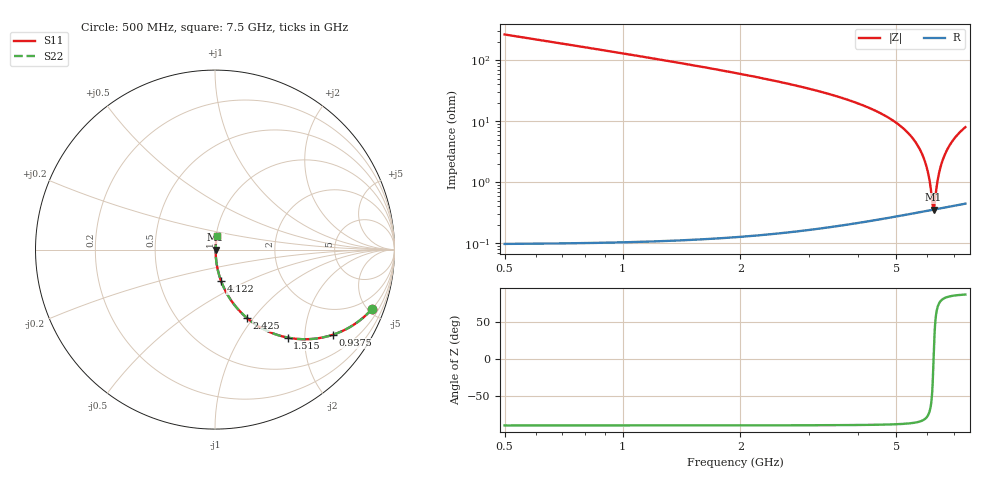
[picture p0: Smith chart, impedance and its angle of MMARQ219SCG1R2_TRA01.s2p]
! MMARQ219SCG1R2_TRA01  S-PARAMETER MODEL  ( General Type )
! Model Generated by TAIYO YUDEN Corporation (http://www.ty-top.com)
! Version 1.0
! TAIYO YUDEN Control No. 180601
! Copyright(c) 2018 TAIYO YUDEN CO.,LTD. All Rights Reserved.
! Product Description (link to TY-COMPAS)
! https://ds.yuden.co.jp/TYCOMPAS/or/detail?pn=MMARQ219SCG1R2BTRA01&u=M
! Products Name : Multilayer Ceramic Capacitors
! Characteristics :
!  Capacitance : 1.2 pF , Rated Voltage : 250V , TCC : CG / C0G
!  Case Size : 2.0 x 1.25 / 0.079 x 0.049 [mm/inch] , Thickness : 0.85 / 0.033 [mm/inch]
!  (Conditions: Temperature = 25 degC , DC Bias Current/Voltage = 0A / 0V)
! External Node Assignments :
!  1  o---| |---o  2
! GND o---------o GND
! Frequency Range : 500MHz  -  7500MHz  [ 401 STEP ]
# MHz S RI R 50
! Freq[MHz].  S11 Real  S11 Imag  S21 Real  S21 Imag  S12 Real  S12 Imag  S22 Real  S22 Imag
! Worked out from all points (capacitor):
!   401 points, 500 MHz to 7.5 GHz, reference 50 ohm
!   read as one part in series: C = 1.2 pF near 535 MHz
!   lowest |Z| = 354 mohm at 6.223 GHz (marker M1)
!   series resonance near 6.222 GHz, so ESL is about 550 pH
!   S11 on the Smith chart (normalised r, x): 500 MHz: 1.00, -5.27; 937.5 MHz: 1.00, -2.76; 1.515 GHz: 1.00, -1.65; 2.425 GHz: 1.00, -0.93; 4.122 GHz: 1.00, -0.36; 7.5 GHz: 1.01, +0.16
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500  0.874 -0.3316  0.126 0.3316  0.126 0.3316  0.874 -0.3316
937.5  0.6564 -0.4745  0.3436 0.4745  0.3436 0.4745  0.6564 -0.4745
1515  0.4041 -0.49  0.5959 0.49  0.5959 0.49  0.4041 -0.49
1672.5  0.3512 -0.4766  0.6488 0.4766  0.6488 0.4766  0.3512 -0.4766
2425  0.1776 -0.3806  0.8224 0.3806  0.8224 0.3806  0.1776 -0.3806
2845  0.1205 -0.3234  0.8795 0.3234  0.8795 0.3234  0.1205 -0.3234
4000  0.0382 -0.1863  0.9618 0.1863  0.9618 0.1863  0.0382 -0.1863
4122.5  0.0334 -0.1737  0.9666 0.1737  0.9666 0.1737  0.0334 -0.1737
5172.5  0.00897 -0.078  0.991 0.078  0.991 0.078  0.00897 -0.078
5592.5  0.00514 -0.045  0.9949 0.045  0.9949 0.045  0.00514 -0.045
5872.5  0.00389 -0.0243  0.9961 0.0243  0.9961 0.0243  0.00389 -0.0243
6047.5  0.00356 -0.012  0.9964 0.012  0.9964 0.012  0.00356 -0.012
6100  0.00352 -0.00831  0.9965 0.00831  0.9965 0.00831  0.00352 -0.00831
6187.5  0.00351 -0.00231  0.9965 0.00231  0.9965 0.00231  0.00351 -0.00231
6222.5  0.00353 6.66e-05  0.9965 -6.66e-05  0.9965 -6.66e-05  0.00353 6.66e-05
6257.5  0.00356 0.00243  0.9964 -0.00243  0.9964 -0.00243  0.00356 0.00243
6345  0.00368 0.00828  0.9963 -0.00828  0.9963 -0.00828  0.00368 0.00828
6415  0.00383 0.0129  0.9962 -0.0129  0.9962 -0.0129  0.00383 0.0129
6502.5  0.00407 0.0186  0.9959 -0.0186  0.9959 -0.0186  0.00407 0.0186
6730  0.00498 0.0331  0.995 -0.0331  0.995 -0.0331  0.00498 0.0331
7062.5  0.00697 0.0533  0.993 -0.0533  0.993 -0.0533  0.00697 0.0533
7500  0.0106 0.0785  0.9894 -0.0785  0.9894 -0.0785  0.0106 0.0785
